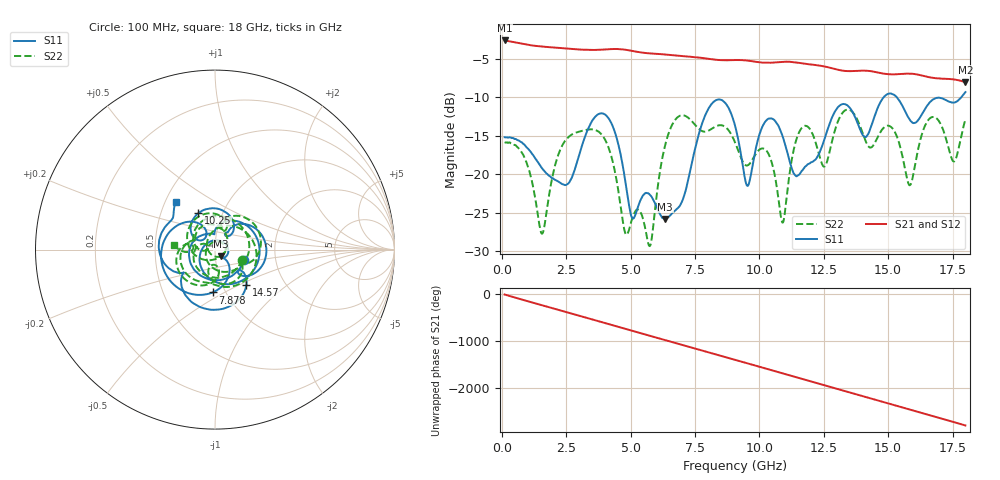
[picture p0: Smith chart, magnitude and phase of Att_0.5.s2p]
#  HZ  S  DB  R  50.00
! Rohde & Schwarz Vector Network Analyzer
! Rohde-Schwarz,ZNB40-4Port,1311601084101679,3.45
! Created: UTC 4/25/2025, 8:41:22 AM
! freq[Hz]  db:S11  ang:S11  db:S21  ang:S21  db:S12  ang:S12  db:S22  ang:S22
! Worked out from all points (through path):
!   1750 points, 100 MHz to 18 GHz, reference 50 ohm
!   highest |S21| = -2.57 dB at 100 MHz (marker M1); lowest = -8.0 dB at 18 GHz (marker M2)
!   group delay of S21, straight-line fit = 428 ps
!   lowest |S11| = -25.9 dB at 6.333 GHz (marker M3), VSWR 1.11, Z = 53.4 - j4.06 ohm
!   |S11| at or under -10 dB: start of sweep to 14.82 GHz; 15.34 GHz to 17.84 GHz (2.495 GHz wide, 15 % of centre)
!   |S22| runs from -29.4 to -11.6 dB; largest |S21 - S12| = 0.0011
!   S11 on the Smith chart (normalised r, x): 100 MHz: 1.38, -0.17; 7.878 GHz: 0.87, -0.44; 10.25 GHz: 0.77, +0.33; 14.57 GHz: 1.29, -0.55; 18 GHz: 0.57, +0.34
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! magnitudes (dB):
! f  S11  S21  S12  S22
! 100 MHz  -15.2  -2.6  -2.6  -15.8
! 1.553 GHz  -19.2  -3.4  -3.4  -27.8
! 2.229 GHz  -21.1  -3.6  -3.6  -17.1
! 3.088 GHz  -16.5  -3.8  -3.8  -14.4
! 4.04 GHz  -12.3  -3.7  -3.7  -15.8
! 4.828 GHz  -21.8  -3.8  -3.8  -27.9
! 5.749 GHz  -22.7  -4.3  -4.3  -29.3
! 6.067 GHz  -24.7  -4.3  -4.3  -21.2
! 6.333 GHz  -25.9  -4.4  -4.4  -16.3
! 7.878 GHz  -12.4  -4.9  -4.9  -14.5
! 9.055 GHz  -13.7  -5.1  -5.1  -15.9
! 9.536 GHz  -21.5  -5.2  -5.2  -18.9
! 10.25 GHz  -13.0  -5.5  -5.5  -16.9
! 10.91 GHz  -15.1  -5.4  -5.4  -26.3
! 11.46 GHz  -20.2  -5.5  -5.5  -15.2
! 12.04 GHz  -18.4  -5.7  -5.7  -14.6
! 14.57 GHz  -11.5  -6.7  -6.7  -15.3
! 15.02 GHz  -9.5  -7.0  -7.0  -13.7
! 15.84 GHz  -12.9  -6.9  -6.9  -21.4
! 16.59 GHz  -10.7  -7.4  -7.4  -12.8
! 17.55 GHz  -10.7  -7.6  -7.7  -18.3
! 18 GHz  -9.3  -8.0  -8.0  -12.9
